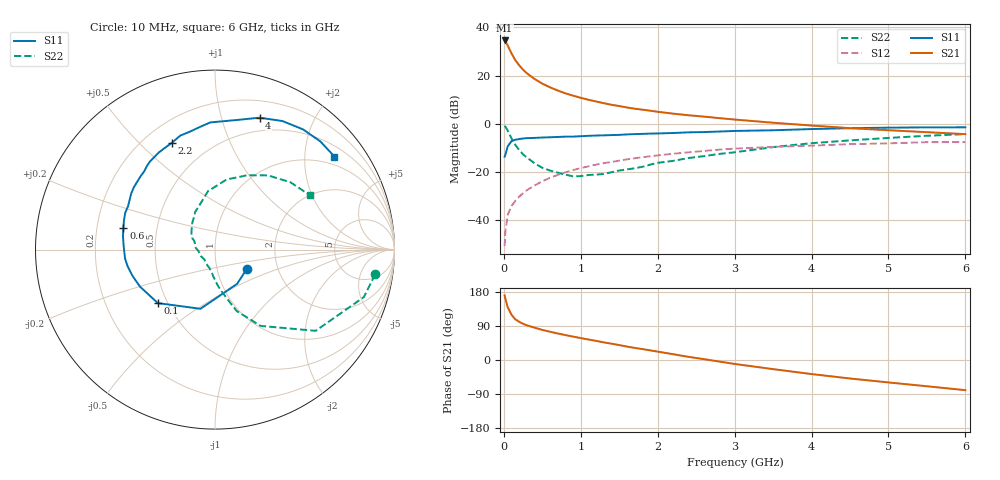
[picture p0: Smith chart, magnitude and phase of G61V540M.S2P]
! SIEMENS Small Signal Semiconductors
! BFG193
! Si NPN RF Bipolar Junction Transistor in SOT223
! VCE = 1.5 V  IC = 40 mA
! Common Emitter S-Parameters:  August  1996
# GHz  S  MA  R  50
!  f  S11  S21  S12  S22
! GHz  MAG  ANG  MAG  ANG  MAG  ANG  MAG  ANG
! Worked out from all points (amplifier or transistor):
!   36 points, 10 MHz to 6 GHz, reference 50 ohm
!   highest |S21| = 34.5 dB at 10 MHz (marker M1)
!   |S21| within 3 dB of that: start of sweep to 63.89 MHz
!   unconditionally stable (mu >= 1): 391 MHz to 2.68 GHz
!   at 250 MHz: K = 0.91, MSG = 25.6 dB, |S12| = -28.8 dB
!   at 1.4 GHz: K = 1.06, MAG = 10.3 dB, |S12| = -15.8 dB
!   at 6 GHz: K = 0.95, MSG = 1.6 dB, |S12| = -7.6 dB
!   S11 on the Smith chart (normalised r, x): 10 MHz: 1.39, -0.32; 100 MHz: 0.44, -0.33; 600 MHz: 0.32, +0.10; 2.2 GHz: 0.31, +0.63; 4 GHz: 0.36, +1.33; 6 GHz: 0.76, +2.73
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0.01  0.2075 -31.8  53.28 170.2  0.0029 87.8  0.9029 -8.8
0.02  0.2271 -57.2  51 161.7  0.0058 81.2  0.8705 -17.7
0.05  0.3396 -103.8  41.92 139.4  0.0129 67.1  0.7206 -38.9
0.1  0.4363 -136.9  28.67 119.3  0.0198 63.0  0.4954 -59.1
0.15  0.4662 -153.8  20.72 107.4  0.0253 61.5  0.3638 -70.5
0.2  0.4821 -162.2  16.21 100.7  0.0308 63.7  0.2859 -75.8
0.25  0.4954 -169.1  13.18 95.5  0.0363 64.3  0.2315 -81.6
0.3  0.5036 -174.3  11.12 91.5  0.042 65.1  0.1992 -85.8
0.4  0.5088 178.2  8.453 85.3  0.0527 65.9  0.151 -93.4
0.5  0.518 171.8  6.787 79.4  0.0641 64.8  0.1224 -100.0
0.6  0.5246 166.8  5.691 74.6  0.076 64.2  0.1073 -107.0
0.7  0.5326 162.2  4.892 70.0  0.0868 62.9  0.097 -116.3
0.8  0.5405 157.7  4.274 65.8  0.0983 60.9  0.088 -126.4
1.1  0.5622 146.1  3.14 54.0  0.1311 55.5  0.0866 -154.3
1.6  0.6015 129.0  2.173 35.5  0.1829 44.2  0.1131 168.1
2.2  0.6426 111.8  1.621 15.3  0.2389 30.1  0.1697 140.3
2.8  0.69 96.6  1.308 -4.1  0.2907 15.6  0.2366 118.0
3.5  0.7324 80.4  1.05 -24.1  0.3316 -2.1  0.328 96.8
4  0.776 71.3  0.918 -37.1  0.3517 -11.9  0.3959 80.6
4.5  0.8089 62.3  0.809 -48.8  0.378 -21.9  0.4518 66.5
5.5  0.8412 45.8  0.669 -69.3  0.4152 -44.6  0.5636 41.7
6  0.8437 37.9  0.609 -79.6  0.4167 -57.6  0.61 29.7
